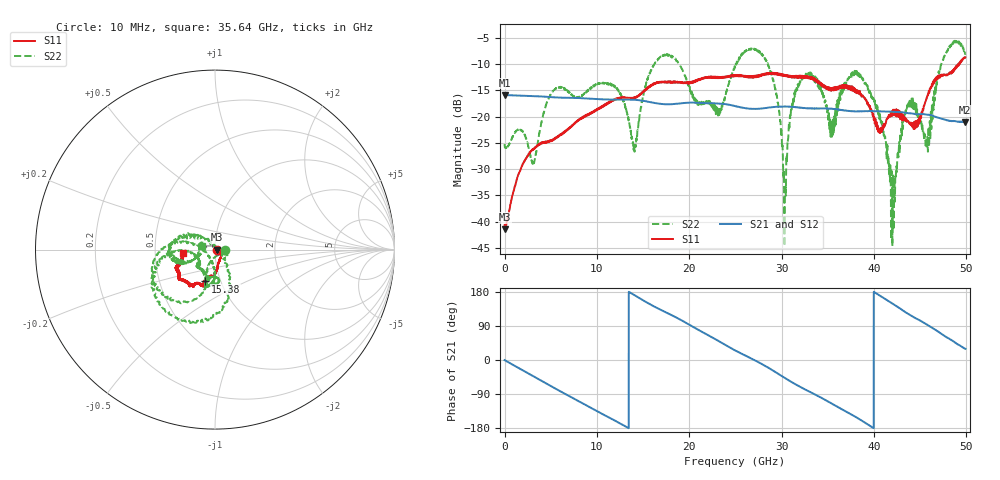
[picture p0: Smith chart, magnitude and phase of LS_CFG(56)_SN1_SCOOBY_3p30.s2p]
!Keysight Technologies,N5245B,MY58422026,A.13.80.08
!Date: Thursday, March 19, 2020 23:44:29
!Correction: S11(Full 2 Port(1,2))
!S21(Full 2 Port(1,2))
!S12(Full 2 Port(1,2))
!S22(Full 2 Port(1,2))
!S2P File: Measurements: S11, S21, S12, S22:
# Hz S DB R 50.0
!freq dBS11 angS11 dBS21 angS21 dBS12 angS12 dBS22 angS22
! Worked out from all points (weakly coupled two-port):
!   4991 points, 10 MHz to 49.91 GHz, reference 50 ohm
!   highest |S21| = -15.90 dB at 10 MHz (marker M1); lowest = -21.1 dB at 49.82 GHz (marker M2)
!   lowest |S11| = -41.4 dB at 30 MHz (marker M3), VSWR 1.02, Z = 50.9 - j0.0333 ohm
!   |S11| at or under -10 dB: start of sweep to 49.13 GHz; 49.15463 GHz to 49.23102 GHz (76.39 MHz wide, 0.155 % of centre)
!   |S22| runs from -44.6 to -5.5 dB; largest |S21 - S12| = 0.0016
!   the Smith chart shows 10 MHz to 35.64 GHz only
!   S11 on the Smith chart (normalised r, x): 10 MHz: 1.02, -0.01; 15.38 GHz: 0.84, -0.31; 35.64 GHz: 0.70, -0.02
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1e7  -40.62 -17.9  -15.90 -0.3  -15.89 -0.3  -25.23 0.5
3e7  -41.44 -2.2  -15.91 -0.5  -15.90 -0.5  -25.76 -2.3
8.33e9  -20.42 -81.2  -16.51 -113.1  -16.51 -113.0  -16.07 -99.3
1.204e10  -16.73 -91.4  -16.78 -161.1  -16.78 -161.1  -14.45 -96.0
1.407e10  -16.47 -99.9  -16.82 171.2  -16.82 171.3  -26.43 -143.7
1.538e10  -14.61 -107.6  -17.12 152.2  -17.11 152.3  -13.55 169.9
1.665e10  -13.56 -108.1  -17.53 135.7  -17.53 135.8  -9.08 -167.2
2.312e10  -12.69 -121.7  -17.51 51.0  -17.51 51.2  -19.81 -149.0
2.496e10  -12.28 -126.2  -17.99 25.5  -17.98 25.7  -10.59 -169.2
2.854e10  -11.95 -139.0  -18.31 -19.9  -18.31 -19.7  -10.23 -79.2
3.037e10  -12.27 -144.9  -18.10 -47.5  -18.10 -47.3  -33.99 39.4
3.135e10  -12.42 -150.4  -18.18 -61.8  -18.19 -61.5  -16.61 146.8
3.328e10  -12.69 -157.3  -18.44 -86.9  -18.45 -86.5  -12.03 -169.3
3.564e10  -15.02 -175.4  -18.53 -117.9  -18.47 -117.4  -23.20 158.1
3.839e10  -15.63 174.4  -19.03 -155.5  -18.97 -155.7  -11.68 -163.4
4.16e10  -19.81 103.0  -19.07 155.4  -19.09 155.3  -28.52 66.5
4.208e10  -18.70 100.6  -19.10 147.9  -19.12 147.9  -31.30 167.2
4.4e10  -21.13 70.5  -19.40 117.3  -19.41 117.4  -16.90 -38.7
4.577e10  -16.25 6.1  -19.66 93.1  -19.68 93.2  -24.95 109.5
4.675e10  -12.55 5.1  -20.11 78.4  -20.13 78.6  -13.57 -135.7
4.982e10  -8.82 -16.5  -21.10 30.5  -21.11 30.6  -7.43 -13.7
4.991e10  -8.75 -15.6  -21.08 29.4  -21.10 29.4  -8.06 -13.9
